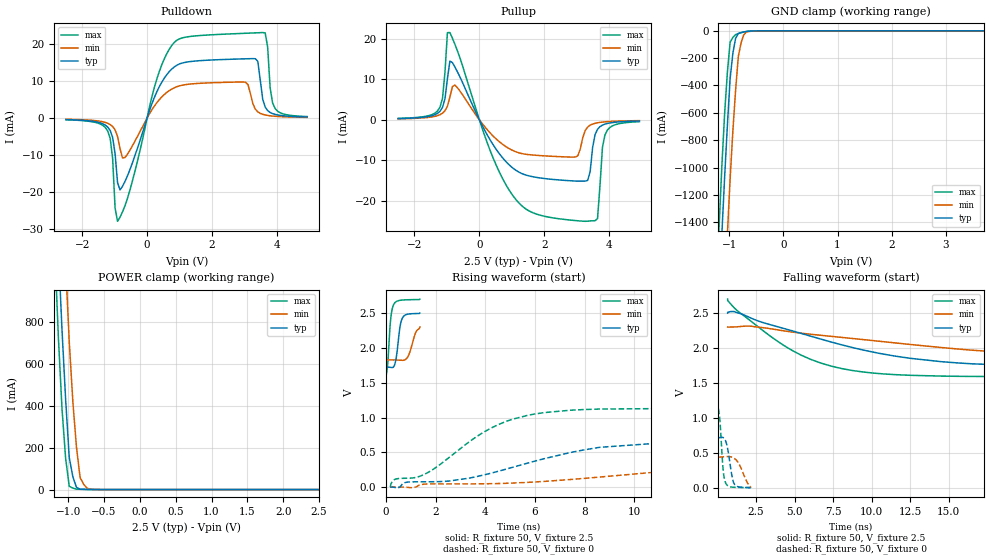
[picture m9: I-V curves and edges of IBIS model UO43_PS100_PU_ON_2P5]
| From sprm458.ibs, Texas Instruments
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|IDG09_OUO43_PS100_PU_OFF_2P75; BUFFER IN NORMAL MODE WITH PULLUP
| OFF
|   Model Cell UO43_PS100_PU_ON_2P5
|IDG09_OUO43_PS100_PU_ON_2P5
[Model]   UO43_PS100_PU_ON_2P5
Model_type   I/O
Polarity   Non-Inverting
Enable   Active-Low
Vinl =  0.7V
Vinh =  1.7V
Cref =  15pF
Rref =  100.00M
Vref =  0V
Vmeas =  1.25
C_comp   1.5511998p   1.5059002p   1.6661999p
[Model Spec]
Vinl   0.7V   0.7V   0.7V
Vinh   1.7V   1.7V   1.7V
[Temperature Range]   25   125   -40
[Voltage Range]   2.5   2.3   2.7
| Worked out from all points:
|   slope of the pulldown table from 0 to 0.375 V, typ, clamps not added: 44.4 ohm
|   slope of the pullup table from 0 to 0.375 V, typ, clamps not added: 67.8 ohm
|   GND clamp passes 1 mA (typ) near -0.57 V on its own axis
|   POWER clamp passes 1 mA (typ) near -0.77 V on its own axis
|   rising waveform, R_fixture 50, V_fixture 2.5: 20-80 % time 166ps typ, 238ps min, 133ps max; typ from 1.72 V to 2.5 V
|   rising waveform, R_fixture 50, V_fixture 0: 20-80 % time 5.05ns typ, 9.63ns min, 2.82ns max; typ from 0.001 V to 0.713 V
|   falling waveform, R_fixture 50, V_fixture 2.5: 20-80 % time 8.45ns typ, 14.1ns min, 4.75ns max; typ from 2.5 V to 1.72 V
|   falling waveform, R_fixture 50, V_fixture 0: 20-80 % time 313ps typ, 532ps min, 204ps max; typ from 0.713 V to 0.001 V
[POWER_clamp]
|   voltage   I(typ)   I(min)   I(max)
-2.5V     14.14A     14.81A     13.77A
-1.187V   1.576A     2.321A     1.148A
-1.136V   1.147A     1.885A     727.1mA
-1.086V   762.4mA    1.471A     386.2mA
-1.035V   430.9mA    1.078A     149.2mA
-984.8mV  152.8mA    706.5mA    15.95mA
-934.3mV  60.92mA    418.4mA    6.9mA
-883.8mV  10.59mA    202mA      2.063mA
-833.3mV  1.805mA    57.47mA    1.446mA
-782.8mV  1.099mA    24.42mA    1.105mA
-732.3mV  637.4uA    5.687mA    800.4uA
2.5V      -62.22uA   -38.43uA   -107.1uA
[Pulldown]
|   voltage   I(typ)   I(min)   I(max)
-2.5V     -396.2uA   -305.7uA   -440.7uA
-1.212V   -2.416mA   -1.384mA   -3.474mA
-1.061V   -5.189mA   -2.255mA   -10.87mA
-909.1mV  -17.44mA   -4.974mA   -27.86mA
-681.8mV  -17.13mA   -10.66mA   -23.68mA
303mV     7.158mA    4.194mA    10.64mA
984.8mV   14.58mA    8.68mA     21.35mA
3.03V     16.01mA    9.688mA    22.91mA
3.333V    16.04mA    2.419mA    23.01mA
3.636V    2.972mA    843.8uA    23mA
3.939V    1.009mA    493.8uA    2.614mA
4.924V    304.5uA    206.1uA    415.7uA
[Pullup]
|   voltage   I(typ)   I(min)   I(max)
-2.5V     313.5uA    255.7uA    361.5uA
-1.212V   2.129mA    1.281mA    3.17mA
-984.8mV  10.18mA    3.39mA     21.48mA
-909.1mV  14.47mA    5.593mA    21.51mA
-757.6mV  13.07mA    8.592mA    18.68mA
984.8mV   -11.57mA   -7.382mA   -18.14mA
2.955V    -15.07mA   -9.137mA   -24.8mA
3.258V    -15.08mA   -2.636mA   -24.98mA
3.636V    -2.316mA   -715uA     -24.31mA
3.788V    -1.293mA   -543uA     -6.805mA
3.939V    -883.6uA   -436.4uA   -2.521mA
4.924V    -281.2uA   -189.2uA   -442.4uA
[GND_clamp]
|   voltage   I(typ)   I(min)   I(max)
-2.5V     -14.52A    -15.32A    -14.07A
-1.187V   -1.916A    -2.778A    -1.414A
-1.136V   -1.475A    -2.331A    -979.6mA
-1.086V   -1.065A    -1.901A    -600.3mA
-1.035V   -689mA     -1.484A    -301.5mA
-984.8mV  -347.4mA   -1.082A    -83.14mA
-934.3mV  -163.7mA   -731.6mA   -48.48mA
-883.8mV  -54.31mA   -433.3mA   -27.35mA
-833.3mV  -19.17mA   -187mA     -19.75mA
-782.8mV  -12.95mA   -87.89mA   -13.95mA
-631.3mV  -2.653mA   -4.727mA   -2.327mA
5V        0A         0A         0A
[Ramp]
| variable   typ   min   max
dV/dt_f 0.47937176/8.5891642n 0.29208734/14.135243n 0.68509636/4.8307861n
dV/dt_r 0.43373437/5.1279352n 0.26921764/9.6469787n 0.68681585/2.845951n
R_load = 50
[Rising Waveform]
R_fixture = 50
V_fixture = 2.5
V_fixture_min = 2.3
V_fixture_max = 2.7
|   time   V(typ)   V(min)   V(max)
0s        1.724V     1.827V     1.591V
70.8ps    1.724V     1.827V     1.813V
175.8ps   1.72V      1.827V     2.39V
292.8ps   1.725V     1.827V     2.614V
393.1ps   1.834V     1.826V     2.662V
549.7ps   2.283V     1.824V     2.682V
650.8ps   2.425V     1.822V     2.687V
895.1ps   2.486V     1.888V     2.691V
1.185ns   2.493V     2.215V     2.693V
1.359ns   2.5V       2.3V       2.7V
[Rising Waveform]
R_fixture = 50
V_fixture = 0
V_fixture_min = 0
V_fixture_max = 0
|   time   V(typ)   V(min)   V(max)
163.6ps   1.277mV    1.03mV     1.705mV
369.6ps   -4.657mV   1.238mV    114.6mV
827.1ps   71.24mV    -1.429mV   128.6mV
1.708ns   78.05mV    46.3mV     215.4mV
4.185ns   197.3mV    50.34mV    840.8mV
5.113ns   287mV      59.57mV    977.6mV
6.351ns   408mV      82.58mV    1.07V
8.602ns   572.2mV    145.5mV    1.122V
13.38ns   693.4mV    293.6mV    1.134V
22.9ns    713.4mV    441.4mV    1.135V
[Falling Waveform]
R_fixture = 50
V_fixture = 2.5
V_fixture_min = 2.3
V_fixture_max = 2.7
|   time   V(typ)   V(min)   V(max)
653.2ps   2.5V       2.3V       2.7V
959.7ps   2.523V     2.301V     2.604V
1.346ns   2.502V     2.305V     2.523V
2.222ns   2.424V     2.312V     2.375V
4.592ns   2.262V     2.237V     1.998V
5.997ns   2.173V     2.199V     1.843V
8.04ns    2.047V     2.153V     1.707V
11.52ns   1.885V     2.074V     1.62V
14.52ns   1.806V     2.008V     1.599V
25.65ns   1.724V     1.827V     1.591V
[Falling Waveform]
R_fixture = 50
V_fixture = 0
V_fixture_min = 0
V_fixture_max = 0
|   time   V(typ)   V(min)   V(max)
59.76ps   713.4mV    441.4mV    1.135V
165.1ps   721.2mV    441.4mV    927mV
361.1ps   719.8mV    444.8mV    260.1mV
424.1ps   708mV      446mV      150.9mV
506.2ps   678.4mV    447.4mV    81.23mV
641.7ps   575mV      449mV      34.69mV
936.4ps   167.6mV    439.6mV    11.73mV
1.072ns   61.33mV    424.4mV    9.408mV
1.387ns   13.89mV    345.4mV    6.993mV
2.158ns   1.277mV    1.03mV     1.705mV
